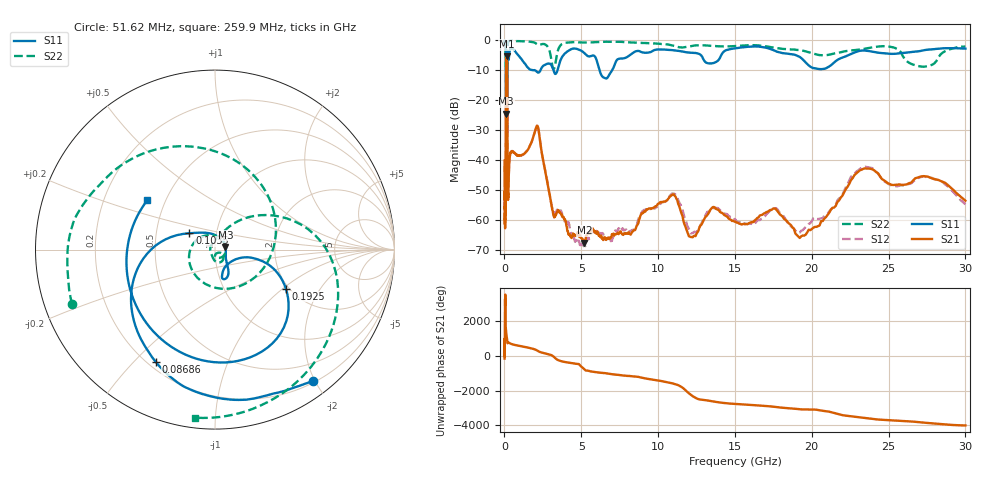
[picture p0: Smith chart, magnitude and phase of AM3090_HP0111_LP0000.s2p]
! Date/Time: Thu, Feb 28, 2019 2:00 PM
! Network Analyzer: Agilent Technologies E8364B Rev: A.07.50.67
! Sweep from 0.010 to 30.000 GHz, 1601 Points, Sweep Type: LOG
! Power Supply: 5.023 V, 0.002 A
# Hz S DB R 50
!freq MagS11 AngS11 MagS21 AngS21 MagS12 AngS12 MagS22 AngS22
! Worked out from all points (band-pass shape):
!   1601 points, 10 MHz to 30 GHz, reference 50 ohm
!   highest |S21| = -5.40 dB at 141.8 MHz (marker M1); lowest = -67.4 dB at 5.206 GHz (marker M2)
!   |S21| within 3 dB of the highest: 111.5 MHz to 175.8 MHz (64.28 MHz wide, 44.8 % of centre)
!   lowest |S11| = -24.5 dB at 109.9 MHz (marker M3), VSWR 1.13, Z = 56.1 + j1.63 ohm
!   |S11| at or under -10 dB: 1.817 GHz to 2.35 GHz (532.5 MHz wide, 25.6 % of centre); 3.187 GHz to 3.455 GHz (269 MHz wide, 8.1 % of centre); 6.185 GHz to 7.011 GHz (825.7 MHz wide, 12.5 % of centre)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
!   |S22| runs from -32.9 to -0.1 dB; largest |S21 - S12| = 0.018
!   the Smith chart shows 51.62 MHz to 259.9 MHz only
!   S11 on the Smith chart (normalised r, x): 51.62 MHz: 0.23, -1.97; 86.86 MHz: 0.23, -0.58; 103.5 MHz: 0.74, +0.14; 192.5 MHz: 1.93, -1.05; 259.9 MHz: 0.40, +0.28
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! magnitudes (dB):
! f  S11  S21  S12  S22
! 10 MHz  -0.3  -40.1  -41.8  -0.5
! 38.04 MHz  -0.5  -59.4  -59.3  -1.2
! 51.62 MHz  -0.8  -50.4  -51.6  -1.4
! 86.86 MHz  -3.0  -49.6  -49.2  -6.4
! 103.5 MHz  -15.4  -14.9  -14.9  -15.4
! 109.9 MHz  -24.5  -9.1  -9.1  -20.1
! 141.8 MHz  -16.5  -5.4  -5.4  -31.5
! 144.7 MHz  -16.8  -5.4  -5.4  -28.2
! 171.5 MHz  -17.1  -7.4  -7.3  -31.0
! 192.5 MHz  -6.9  -24.1  -24.0  -7.8
! 213.8 MHz  -4.1  -51.4  -51.7  -1.8
! 259.9 MHz  -6.6  -50.2  -49.2  -0.5
! 550.5 MHz  -3.0  -37.2  -37.3  -0.2
! 2.084 GHz  -10.4  -28.8  -28.7  -1.3
! 3.188 GHz  -10.0  -58.4  -57.1  -9.6
! 5.206 GHz  -4.4  -67.4  -68.3  -0.8
! 7.926 GHz  -5.8  -64.5  -63.0  -0.7
! 10.81 GHz  -3.3  -52.0  -51.5  -1.7
! 12.19 GHz  -4.2  -65.5  -64.3  -2.0
! 19.7 GHz  -8.0  -64.0  -61.9  -3.9
! 23.48 GHz  -3.5  -42.7  -42.2  -2.9
! 30 GHz  -2.9  -53.5  -54.7  -2.2
